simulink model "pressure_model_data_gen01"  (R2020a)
settings: Solver=VariableStepAuto  StartTime=0.0  StopTime=tfin  RelTol=1e-3
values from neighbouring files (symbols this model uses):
  Ts = 5    [sisopres.m]

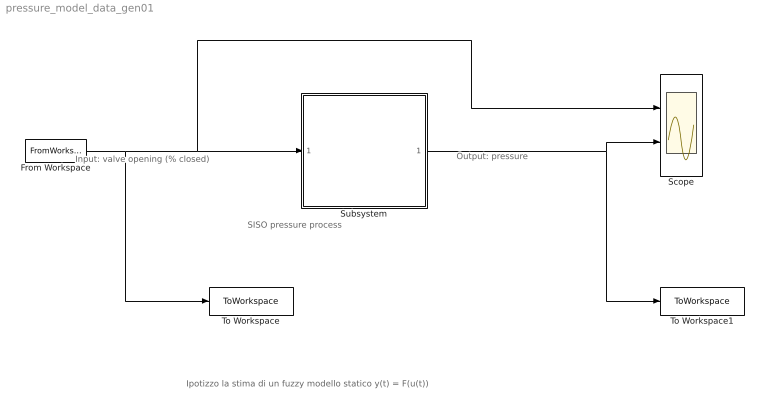
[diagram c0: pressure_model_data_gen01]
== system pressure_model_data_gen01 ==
  note: Ipotizzo la stima di un fuzzy modello statico y(t) = F(u(t))
  note: Output: pressure
  note: Input: valve opening (% closed)
  note: SISO pressure process
  From Workspace : FromWorkspace  VariableName=[tsim U]  SampleTime=Ts
  Scope : Scope  NumInputPorts=2
  Subsystem : Subsystem
  To Workspace : ToWorkspace  VariableName=Psim  SampleTime=Ts
  To Workspace1 : ToWorkspace  VariableName=Tsim  SaveFormat=Timeseries  SampleTime=-1
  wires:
  From Workspace/1 -> To Workspace/1, Scope/1, Subsystem/1(u)
  Subsystem/1(y) -> To Workspace1/1, Scope/2

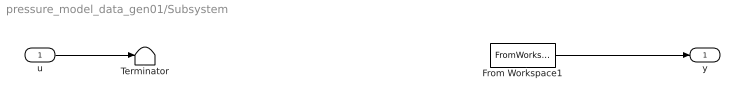
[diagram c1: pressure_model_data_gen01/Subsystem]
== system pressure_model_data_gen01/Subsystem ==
  u : Inport
  From Workspace1 : FromWorkspace  VariableName=[tsim Y]  SampleTime=Ts
  Terminator : Terminator
  y : Outport
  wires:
  From Workspace1/1 -> y/1
  u/1 -> Terminator/1
